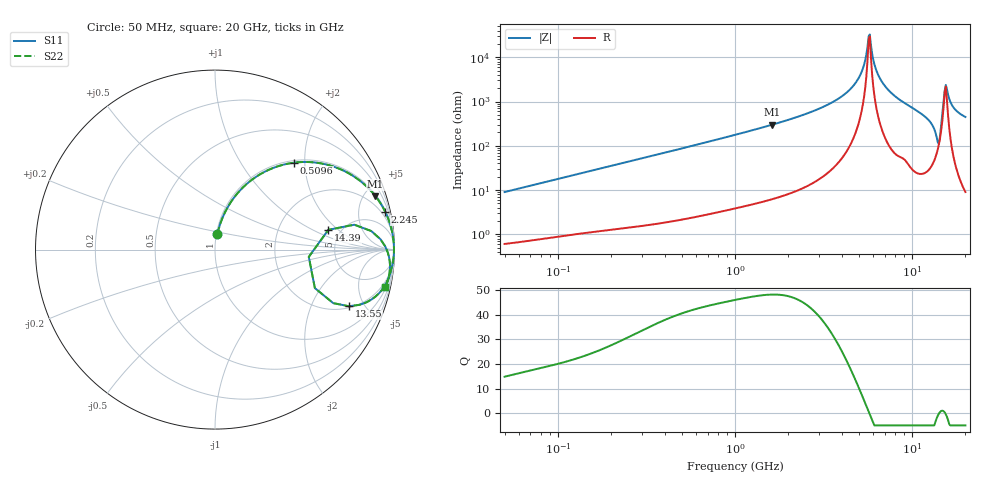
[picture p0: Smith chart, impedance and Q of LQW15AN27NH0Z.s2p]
!Murata Part Number: LQW15AN27NH0Z
!These Parameters are Measured in Series Mode Connection
!  o--[Z]--o
!Port1  Port2
!  o-------o
!Freq. Start=50[MHz] Stop=20[GHz], 401[Steps]
# Hz S RI R 50
!Freq.(Hz) S11(Real) S11(Imag) S21(Real) S21(Imag) S12(Real) S12(Imag) S22(Real) S22(Imag)
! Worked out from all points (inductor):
!   401 points, 50 MHz to 20 GHz, reference 50 ohm
!   read as one part in series: L = 28.5 nH near 51.52 MHz
!   highest Q = 48.3 at 1.615 GHz (marker M1), where L = 29.4 nH
!   self-resonance near 5.683 GHz
!   S11 on the Smith chart (normalised r, x): 50 MHz: 1.01, +0.18; 509.6 MHz: 1.04, +1.77; 2.245 GHz: 1.19, +8.98; 13.55 GHz: 2.10, -3.85; 14.39 GHz: 3.98, +1.49; 20 GHz: 1.18, -8.97
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5e7  0.0139 0.0881  0.9861 -0.0881  0.9861 -0.0881  0.0139 0.0881
1.364002e8  0.0633 0.2226  0.9367 -0.2226  0.9367 -0.2226  0.0633 0.2226
3.721004e8  0.3003 0.445  0.6997 -0.445  0.6997 -0.445  0.3003 0.445
5.096456e8  0.4417 0.4845  0.5583 -0.4845  0.5583 -0.4845  0.4417 0.4845
1e9  0.7525 0.4208  0.2475 -0.4208  0.2475 -0.4208  0.7525 0.4208
1.614971e9  0.8942 0.2974  0.1058 -0.2974  0.1058 -0.2974  0.8942 0.2974
2.245319e9  0.9487 0.2101  0.0513 -0.2101  0.0513 -0.2101  0.9487 0.2101
2.728004e9  0.969 0.162  0.031 -0.162  0.031 -0.162  0.969 0.162
3.792786e9  0.9892 0.0872  0.0108 -0.0872  0.0108 -0.0872  0.9892 0.0872
4.677679e9  0.9953 0.0427  0.00466 -0.0427  0.00466 -0.0427  0.9953 0.0427
5.194772e9  0.9968 0.0208  0.0032 -0.0208  0.0032 -0.0208  0.9968 0.0208
5.683258e9  0.9972 0.0019  0.00276 -0.0019  0.00276 -0.0019  0.9972 0.0019
5.856089e9  0.9972 -0.00443  0.00278 0.00443  0.00278 0.00443  0.9972 -0.00443
6.406762e9  0.9966 -0.0237  0.0034 0.0237  0.0034 0.0237  0.9966 -0.0237
7.442007e9  0.9935 -0.0572  0.00653 0.0572  0.00653 0.0572  0.9935 -0.0572
1.201863e10  0.9377 -0.2141  0.0623 0.2141  0.0623 0.2141  0.9377 -0.2141
1.354865e10  0.7459 -0.3156  0.2541 0.3156  0.2541 0.3156  0.7459 -0.3156
1.438523e10  0.6317 0.1102  0.3683 -0.1102  0.3683 -0.1102  0.6317 0.1102
1.527346e10  0.9484 0.0177  0.0516 -0.0177  0.0516 -0.0177  0.9484 0.0177
1.573793e10  0.9697 -0.0414  0.0303 0.0414  0.0303 0.0414  0.9697 -0.0414
1.721783e10  0.9716 -0.1339  0.0284 0.1339  0.0284 0.1339  0.9716 -0.1339
2e10  0.9488 -0.2106  0.0512 0.2106  0.0512 0.2106  0.9488 -0.2106
